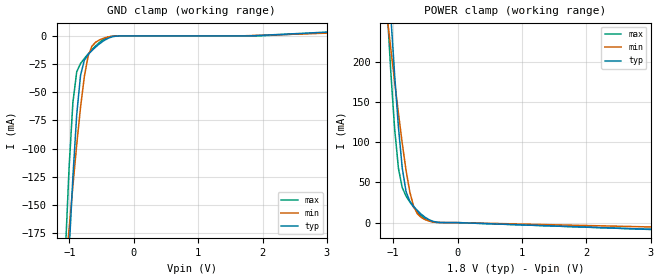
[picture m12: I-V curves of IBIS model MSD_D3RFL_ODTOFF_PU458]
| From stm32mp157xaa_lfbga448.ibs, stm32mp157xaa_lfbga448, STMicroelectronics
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[Model] MSD_D3RFL_ODTOFF_PU458
Model_type   Input
C_comp 2.352pF   2.291pF   2.498pF
Vinh = 1.440V
Vinl = 360.000mV
[Temperature Range]   25.000   125.000   -40.000
[Voltage Range]   1.800V   1.650V   1.950V
[GND Clamp Reference]   0.00V   0.00V   0.00V
[POWER Clamp Reference]   1.800V   1.650V   1.950V
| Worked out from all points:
|   GND clamp passes 1 mA (typ) near -0.34 V on its own axis
|   POWER clamp passes 1 mA (typ) near -0.35 V on its own axis
[GND Clamp]
-1.773V   -1.215A    -712.6mA   -1.314A
-1.064V   -264mA     -211mA     -194mA
-1.005V   -191.5mA   -171.3mA   -117.1mA
-945.5mV  -124.9mA   -132.9mA   -58.89mA
-886.4mV  -69.88mA   -96.53mA   -31.82mA
-827.3mV  -35.06mA   -63.45mA   -24.47mA
-768.2mV  -21.59mA   -36.15mA   -20.07mA
-709.1mV  -16.54mA   -17.88mA   -16.04mA
-650mV    -12.98mA   -9.142mA   -12.24mA
-531.8mV  -6.967mA   -3.536mA   -5.699mA
-236.4mV  -75.02uA   -35.01uA   -7.023uA
3.545V    4.912mA    3.459mA    4.562mA
[Power Clamp]
-1.745V   1.221A     726mA      1.304A
-1.095V   333.9mA    257.3mA    268.4mA
-1.036V   257mA      216.1mA    186.7mA
-977.3mV  184mA      175.6mA    116.9mA
-918.2mV  118.8mA    136.2mA    67.82mA
-859.1mV  68.1mA     98.77mA    43.51mA
-800mV    38.66mA    65.12mA    33.12mA
-740.9mV  26.73mA    38.01mA    25.62mA
-681.8mV  20.18mA    20.17mA    19.08mA
-563.6mV  10.44mA    6.372mA    8.612mA
-268.2mV  161.4uA    99.74uA    32.1uA
3.573V    -9.943mA   -6.426mA   -10.15mA
